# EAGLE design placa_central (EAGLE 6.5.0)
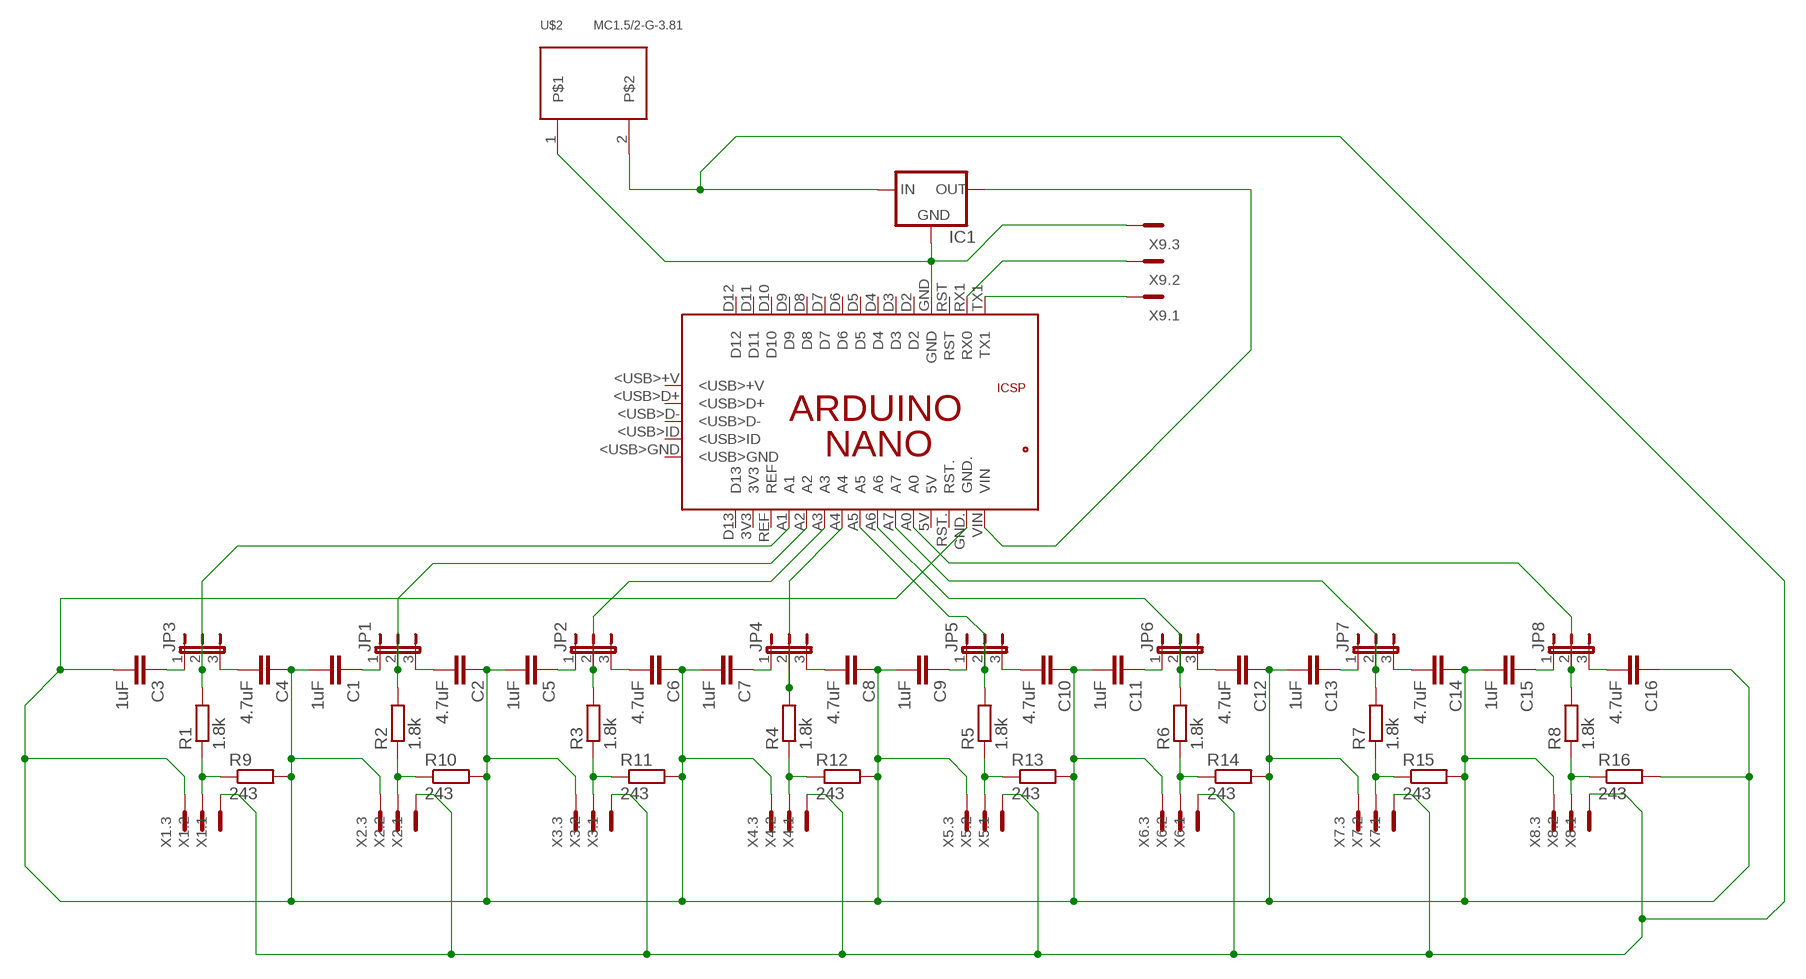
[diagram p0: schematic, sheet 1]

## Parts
C1  1uF  C-EUC1206  [C1206]
C2  4.7uF  C-EUC1206  [C1206]
C3  1uF  C-EUC1206  [C1206]
C4  4.7uF  C-EUC1206  [C1206]
C5  1uF  C-EUC1206  [C1206]
C6  4.7uF  C-EUC1206  [C1206]
C7  1uF  C-EUC1206  [C1206]
C8  4.7uF  C-EUC1206  [C1206]
C9  1uF  C-EUC1206  [C1206]
C10  4.7uF  C-EUC1206  [C1206]
C11  1uF  C-EUC1206  [C1206]
C12  4.7uF  C-EUC1206  [C1206]
C13  1uF  C-EUC1206  [C1206]
C14  4.7uF  C-EUC1206  [C1206]
C15  1uF  C-EUC1206  [C1206]
C16  4.7uF  C-EUC1206  [C1206]
IC1  78XXS  [78XXS]
JP1  JP2E  [JP2]
JP2  JP2E  [JP2]
JP3  JP2E  [JP2]
JP4  JP2E  [JP2]
JP5  JP2E  [JP2]
JP6  JP2E  [JP2]
JP7  JP2E  [JP2]
JP8  JP2E  [JP2]
PCB1  ARDUINO_NANO  [ARDUINO_NANO]
R1  1.8k  R-EU_M1206  [M1206]
R2  1.8k  R-EU_M1206  [M1206]
R3  1.8k  R-EU_M1206  [M1206]
R4  1.8k  R-EU_M1206  [M1206]
R5  1.8k  R-EU_M1206  [M1206]
R6  1.8k  R-EU_M1206  [M1206]
R7  1.8k  R-EU_M1206  [M1206]
R8  1.8k  R-EU_M1206  [M1206]
R9  243  R-EU_M1206  [M1206]
R10  243  R-EU_M1206  [M1206]
R11  243  R-EU_M1206  [M1206]
R12  243  R-EU_M1206  [M1206]
R13  243  R-EU_M1206  [M1206]
R14  243  R-EU_M1206  [M1206]
R15  243  R-EU_M1206  [M1206]
R16  243  R-EU_M1206  [M1206]
U$2  MC1.5/2-G-3.81  [MC1.5/2-G-3.81]
X1  MC3  [MC3]
X2  MC3  [MC3]
X3  MC3  [MC3]
X4  MC3  [MC3]
X5  MC3  [MC3]
X6  MC3  [MC3]
X7  MC3  [MC3]
X8  MC3  [MC3]
X9  MC3  [MC3]

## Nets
GND: C1.2 C2.1 C3.2 C4.1 C5.2 C6.1 C7.2 C8.1 C9.2 C10.1 C11.2 C12.1 C13.2 C14.1 C15.2 C16.1 IC1.GND PCB1.GND PCB1.GND. R9.2 R10.2 R11.2 R12.2 R13.2 R14.2 R15.2 R16.2 U$2.1 X1.3 X2.3 X3.3 X4.3 X5.3 X6.3 X7.3 X8.3 X9.3
N$1: R1.1 R9.1 X1.2
N$3: C4.2 JP3.3
N$4: C3.1 JP3.1
N$5: R2.1 R10.1 X2.2
N$6: PCB1.RX1(RX0) X9.2
N$7: C2.2 JP1.3
N$8: C1.1 JP1.1
N$9: R3.1 R11.1 X3.2
N$10: IC1.OUT PCB1.VIN
N$11: C6.2 JP2.3
N$12: C5.1 JP2.1
N$13: R4.1 R12.1 X4.2
N$14: PCB1.TX1 X9.1
N$15: C8.2 JP4.3
N$16: C7.1 JP4.1
N$17: R5.1 R13.1 X5.2
N$19: C10.2 JP5.3
N$20: C9.1 JP5.1
N$21: R6.1 R14.1 X6.2
N$23: C12.2 JP6.3
N$24: C11.1 JP6.1
N$25: R7.1 R15.1 X7.2
N$27: C14.2 JP7.3
N$28: C13.1 JP7.1
N$29: R8.1 R16.1 X8.2
N$31: C16.2 JP8.3
N$32: C15.1 JP8.1
N$33: JP3.2 PCB1.A1 R1.2
N$34: JP1.2 PCB1.A2 R2.2
N$35: JP2.2 PCB1.A3 R3.2
N$36: JP4.2 PCB1.A4 R4.2
N$37: JP8.2 PCB1.A0 R8.2
N$38: JP7.2 PCB1.A7 R7.2
N$39: JP6.2 PCB1.A6 R6.2
N$40: JP5.2 PCB1.A5 R5.2
N$59: IC1.IN U$2.2 X1.1 X2.1 X3.1 X4.1 X5.1 X6.1 X7.1 X8.1
Unconnected: PCB1.3V3 PCB1.5V PCB1.5V. PCB1.<USB>+V PCB1.<USB>D+ PCB1.<USB>D- PCB1.<USB>GND PCB1.<USB>ID PCB1.D2 PCB1.D3 PCB1.D4 PCB1.D5 PCB1.D6 PCB1.D7 PCB1.D8 PCB1.D9 PCB1.D10 PCB1.D11 PCB1.D12 PCB1.D13 PCB1.GND_ PCB1.MISO PCB1.MOSI PCB1.REF PCB1.RESET.. PCB1.RST PCB1.RST. PCB1.SCK

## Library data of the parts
C1-C16 = resistor:C-EU: CAPACITOR, European symbol
IC1 = v-reg:78XXS: VOLTAGE REGULATOR
JP1-JP8 = jumper:JP2E: JUMPER
PCB1 = E14_Arduino:ARDUINO_NANO: Device for representing an Arduino Nano board with a footprint in an EAGLE design. Created by Dave Young for Element14. More EAGLE documentation at: http://www.element14.com/community/community/knode/cadsoft_eagle
R1-R16 = resistor:R-EU_: RESISTOR, European symbol
U$2 = rpascoal:MC1.5/2-G-3.81
X1-X9 = con-phoenix-381_l:MC3: Mini-Combicon 3.81mm horizontal 3-polig (ohne Gegenstecker)

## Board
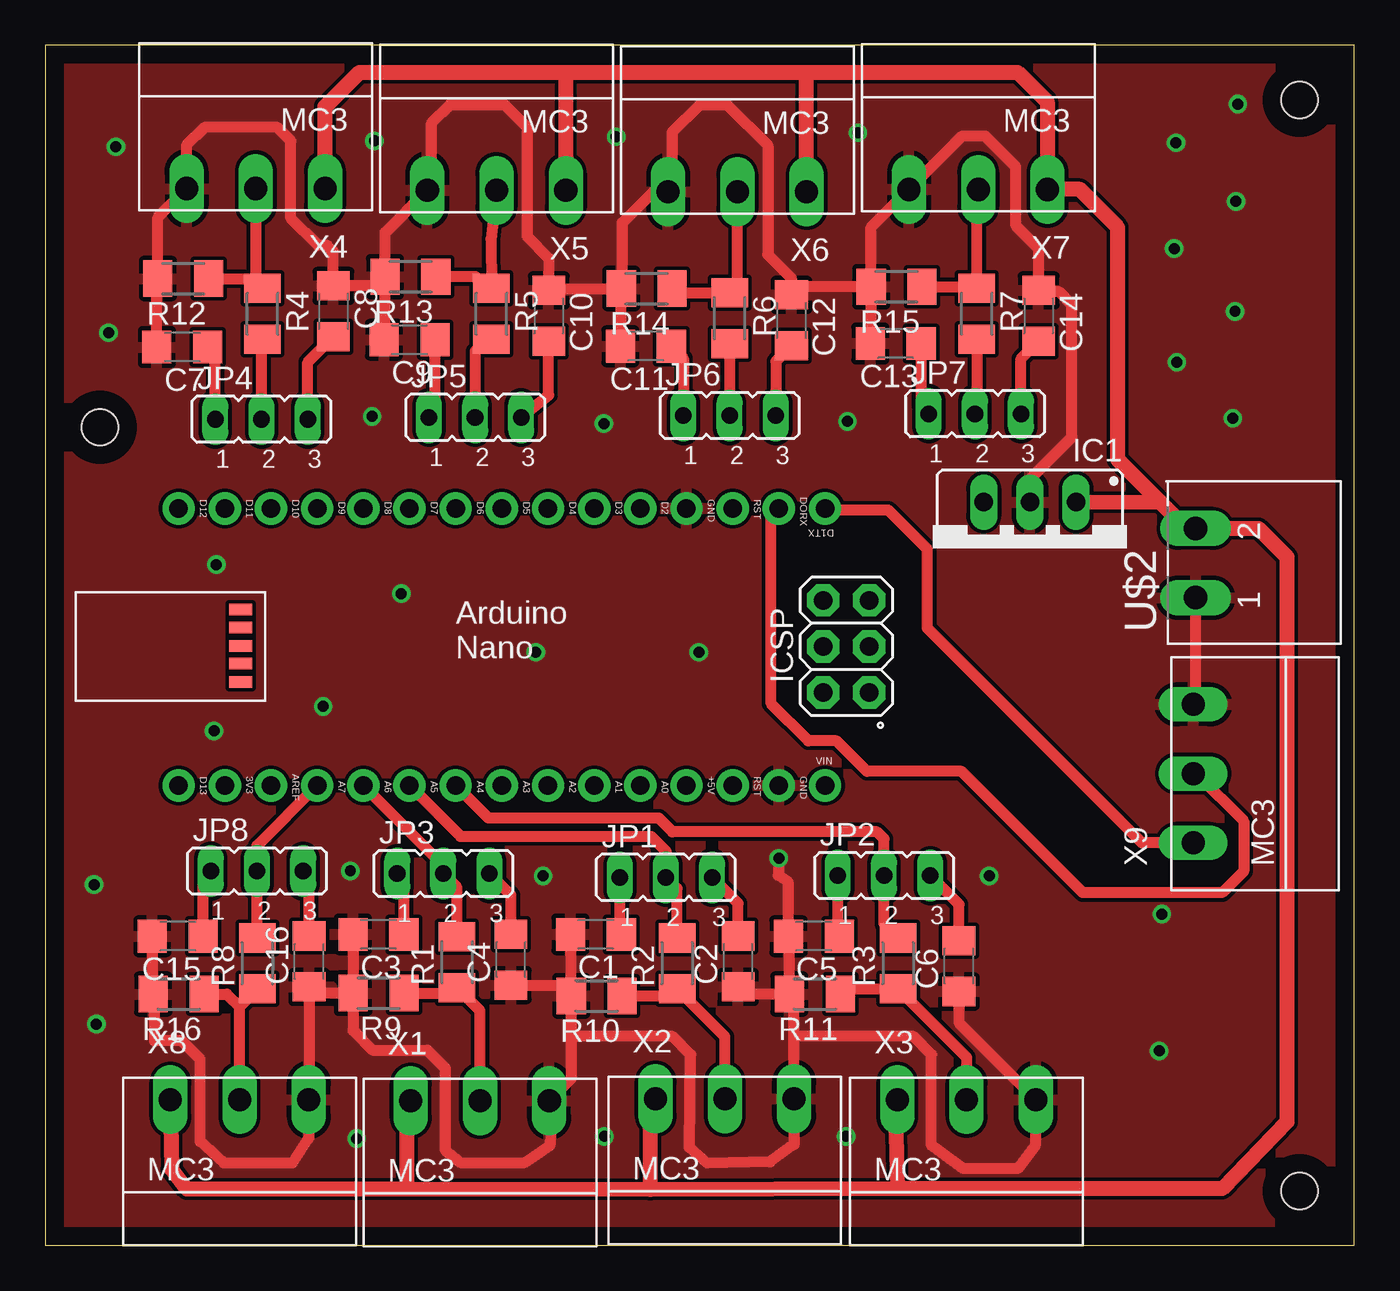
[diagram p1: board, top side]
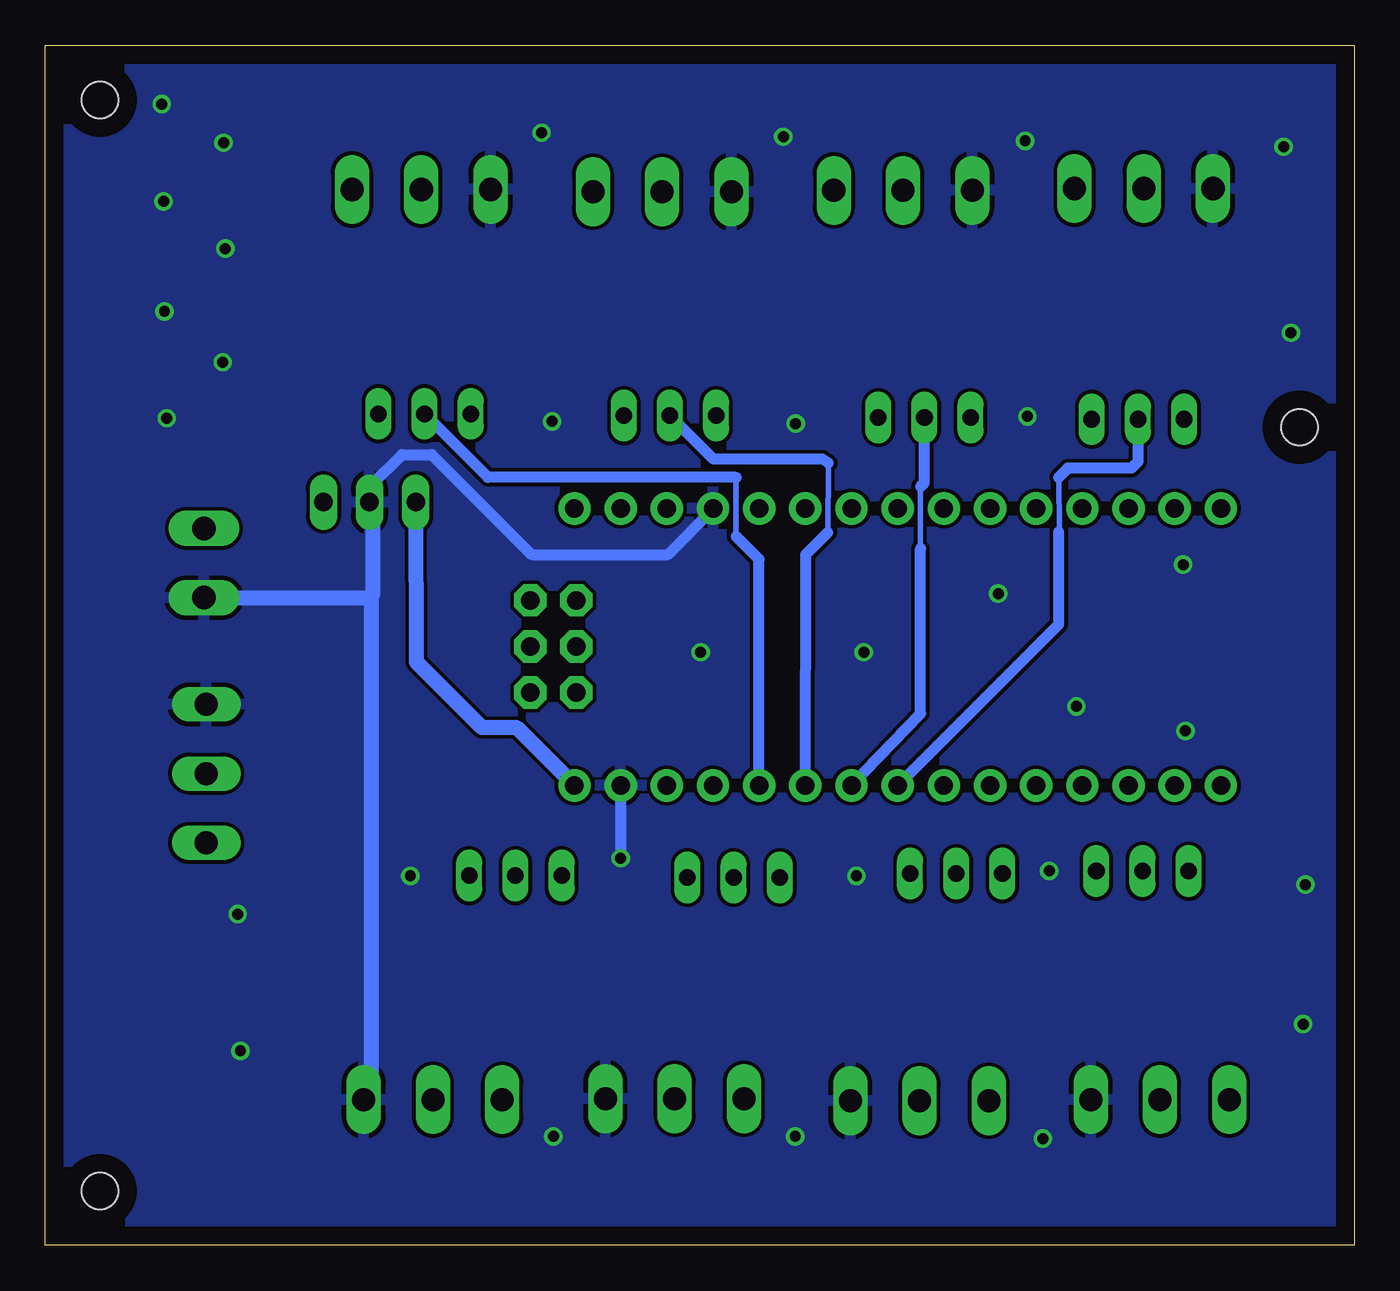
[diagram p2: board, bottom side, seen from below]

Size 72 x 66 mm. Coordinates in mm from the lower left corner, seen from the top.
Outline: 0,0 72,0 72,66 0,66 0,0
Copper layers (1*16): Top 0.035mm / dielectric 1.5mm / Bottom 0.035mm
Design rules "default": minimum track width 8mil, minimum drill 20mil, track to track 8mil, track to pad 8mil, pad to pad 8mil, via to via 10mil, smd to smd 8mil, copper to edge 40mil, drill to drill 8mil, minimum pad ring 10mil, minimum via ring 8mil, stop-mask expansion 4mil, vias tented up to drill 0mil, thermal gap 10mil
Holes 2 mm at 69,63 69,3 3,45

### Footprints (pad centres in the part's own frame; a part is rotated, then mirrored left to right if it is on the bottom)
C1206 = smd 1.6 x 1.8: 1 -1.4,0; 2 1.4,0
78XXS = drill 1.016 long: GND 0,-2.54; IN -2.54,-2.54; OUT 2.54,-2.54
JP2 = drill 0.914 long: 1 -2.54,0; 2 0,0; 3 2.54,0
ARDUINO_NANO = drill 1.016 pad 1.778: 3V3 6.35,1.27; 5V 31.75,1.27; A0 11.43,1.27; A1 13.97,1.27; A2 16.51,1.27; A3 19.05,1.27; A4 21.59,1.27; A5 24.13,1.27; A6 26.67,1.27; A7 29.21,1.27; D2 29.21,16.51; D3 26.67,16.51; D4 24.13,16.51; D5 21.59,16.51; D6 19.05,16.51; D7 16.51,16.51; D8 13.97,16.51; D9 11.43,16.51; D10 8.89,16.51; D11 6.35,16.51; D12 3.81,16.51; D13 3.81,1.27; GND 31.75,16.51; GND. 36.83,1.27; REF 8.89,1.27; RST 34.29,16.51; RST. 34.29,1.27; RX1 36.83,16.51; TX1 39.37,16.51; VIN 39.37,1.27 | drill 1.016 pad 1.778 octagon: 5V. 39.268,6.375; GND_ 39.268,11.455; MISO 41.808,6.375; MOSI 39.268,8.915; RESET.. 41.808,11.455; SCK 41.808,8.915 | smd 1.27 x 0.635: <USB>+V 7.214,10.947; <USB>D+ 7.214,9.957; <USB>D- 7.214,8.941; <USB>GND 7.214,6.96; <USB>ID 7.214,7.976
M1206 = smd 1.6 x 2: 1 -1.4,0; 2 1.4,0
MC1.5/2-G-3.81 = drill 1.3 long: 1 -3.81,8; 2 0,8
MC3 = drill 1.27 long: 1 -3.81,0; 2 0,0; 3 3.81,0

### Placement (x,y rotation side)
C1  30.28,17.11 180 top
C2  38.11,15.62 90 top
C3  18.32,17.11 180 top
C4  25.61,15.72 90 top
C5  42.28,17.01 180 top
C6  50.26,15.37 90 top
C7  7.53,49.41 180 top
C8  15.84,51.38 270 top
C9  20.03,49.81 180 top
C10  27.69,51.13 270 top
C11  33.03,49.46 180 top
C12  41.04,50.88 270 top
C13  46.78,49.61 180 top
C14  54.64,51.13 270 top
C15  7.28,17.01 180 top
C16  14.51,15.62 90 top
IC1  54.16,38.34 180 top
JP1  34.14,20.24 0 top
JP2  46.14,20.34 0 top
JP3  21.89,20.45 0 top
JP4  11.89,45.44 0 top
JP5  23.64,45.54 0 top
JP6  37.64,45.64 0 top
JP7  51.14,45.74 0 top
JP8  11.64,20.59 0 top
PCB1  3.52,24.03 0 top
R1  22.64,15.58 90 top
R2  34.76,15.51 90 top
R3  46.91,15.51 90 top
R4  11.94,51.24 270 top
R5  24.54,51.24 270 top
R6  37.64,50.99 270 top
R7  51.24,51.24 270 top
R8  11.66,15.51 90 top
R9  18.33,13.88 180 top
R10  30.33,13.73 180 top
R11  42.33,13.83 180 top
R12  7.58,53.18 180 top
R13  20.08,53.28 180 top
R14  33.08,52.63 180 top
R15  46.83,52.73 180 top
R16  7.33,13.83 180 top
U$2  71.28,39.44 90 top
X1  23.91,7.96 0 top
X2  37.38,8.07 0 top
X3  50.68,8.02 0 top
X4  11.57,58.13 180 top
X5  24.82,58.03 180 top
X6  38.07,57.95 180 top
X7  51.32,58.08 180 top
X8  10.68,8.02 0 top
X9  63.15,25.95 90 top

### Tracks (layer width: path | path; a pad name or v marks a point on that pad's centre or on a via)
GND  (via drill 0.6)
  Top 0.61: C15.2 5.88,13.88 R16.2 5.93,13.25 6,13.25 6,11.25 7.5,11.25 8.5,10.25 8.5,5.72 9.82,4.53 13.57,4.53 14.49,5.92 X8.3 14.51,9.79 C16.1 14.85,13.88 R9.2 | C3.2 R9.2 | R9.2 16.92,11.83 18,10.75 21,10.75 22,9.75 22,5.25 22.85,4.55 26.35,4.55 27.75,5.5 27.8,6.16 X1.3 28.93,9.18 28.93,11.25 | C1.2 28.88,13.78 R10.2 | R10.2 28.93,11.25 | 28.93,11.25 29.18,11.5 34.5,11.5 35.5,10.5 35.42,5.38 36.4,4.53 39.88,4.6 41.19,5.57 X2.3 41.19,11.5 | 41.19,11.5 41.19,13.57 R11.2 | R11.2 38.5,13.83 C2.1 | R11.2 40.93,16.96 C5.2 40.88,19.97 40.33,20.35 v40.35,21.3 | C4.1 28.34,14.32 R10.2 | 41.19,11.5 47.75,11.5 48.75,10.5 48.75,5.5 50.5,4.22 53.5,4.22 54.49,5.54 X3.3 50.26,12.25 C6.1 | C7.2 6.13,53.13 R12.2 6.18,56.55 X4.3 7.75,60.5 8.75,61.5 12.75,61.5 13.5,60.75 13.5,56.5 15,55 15.5,55 15.84,54.66 C8.1 18.18,52.78 R13.2 | C9.2 18.68,49.86 R13.2 | R13.2 18.68,55.7 X5.3 21.25,58.27 21.25,61.75 22.25,62.75 25.25,62.75 26.5,61.5 26.5,55.5 27.69,54.31 C10.1 27.79,52.63 R14.2 | R14.2 31.63,52.58 C11.2 | R14.2 31.75,52.7 31.75,56.25 33.68,58.18 X6.3 34.5,58.42 34.5,61.25 36,62.75 37.5,62.75 39.75,60.5 39.75,54.5 41.04,53.21 C12.1 41.49,52.73 R15.2 | R15.2 45.43,49.66 C13.2 | R15.2 45.43,56 X7.3 50.45,61.02 51.7,61.02 53.38,59.35 53.38,56.12 54.64,54.86 C14.1 54.72,52.45 55.77,52.45 56.48,51.75 56.48,44.45 54.14,42.12 IC1.GND | X9.3 63.28,29.76 U$2.1
  Bottom 0.61: PCB1.GND 35.27,40.48 37.75,38 45.25,38 50.75,43.5 52.39,43.5 54.14,41.75 IC1.GND | PCB1.GND. v40.35,21.3
  Bottom 0.813: U$2.1 54.15,35.63 54.05,35.73 | IC1.GND 54,40.76 54,35.77 54.05,35.73 | X3.3 54.05,8.46 54.05,35.73
  other vias: 65.6,62.77 65.5,57.42 65.45,51.38 65.33,45.5 62.25,48.58 62.1,54.83 62.2,60.65 61.42,18.23 61.27,10.7 15.28,29.65 19.57,35.85 35.95,32.62 26.98,32.62 9.4,37.45 9.28,28.3 3.88,60.42 3.48,50.2 2.67,19.85 2.8,12.18 44.12,45.33 30.73,45.2 17.98,45.6 27.38,20.32 16.77,20.6 51.92,20.32 44.05,6 30.75,6 17.12,5.88 44.7,61.2 31.4,60.98 18.1,60.75
  pour Bottom: 72.25,66.95 72.25,-0.57 -0.72,-0.57 -0.72,66.95
  pour Top: -1.18,67.7 72.97,67.7 72.97,-1.45 -1.6,-1.45
N$1
  Top 0.61: X1.2 23.91,12.91 R1.1 22.34,13.88 R9.1
N$3
  Top 0.61: C4.2 25.61,19.27 JP3.3
N$4
  Top 0.61: C3.1 19.72,20.08 JP3.1
N$5
  Top 0.61: X2.2 37.38,11.49 R2.1 34.38,13.73 R10.1
N$6
  Top 0.61: X9.2 63.33,25.95 65.92,23.35 65.92,20.57 64.75,19.4 57.08,19.4 50.4,26.07 45.2,26.07 43.52,27.75 41.98,27.75 39.92,29.8 39.92,40.12 PCB1.RX1
N$7
  Top 0.61: C2.2 38.11,18.81 JP1.3
N$8
  Top 0.61: C1.1 31.6,17.11 JP1.1
N$9
  Top 0.61: R11.1 44.01,14.11 R3.1 50.68,10.34 X3.2
N$10
  Bottom 0.813: IC1.OUT 51.6,32.1 48,28.5 46.09,28.5 PCB1.VIN
N$11
  Top 0.61: C6.2 50.26,18.76 JP2.3
N$12
  Top 0.61: C5.1 43.6,17.09 JP2.1
N$13
  Top 0.61: R12.1 11.4,53.18 R4.1 11.57,53.01 X4.2
N$14
  Top 0.61: X9.1 60.34,22.14 48.52,33.95 48.52,38.3 46.38,40.45 42.98,40.45 PCB1.TX1
N$15
  Top 0.61: JP4.3 14.43,48.57 C8.2
N$16
  Top 0.61: JP4.1 9.35,48.99 C7.1
N$17
  Top 0.61: X5.2 24.52,55.35 R5.1 23.65,53.28 R13.1
N$19
  Top 0.61: JP5.3 27.69,46.77 C10.2
N$20
  Top 0.61: JP5.1 21.43,45.87 C9.1
N$21
  Top 0.61: R14.1 34.72,52.39 R6.1 38.07,52.82 X6.2
N$23
  Top 0.61: C12.2 40.18,48.62 JP6.3
N$24
  Top 0.61: C11.1 35.1,48.79 JP6.1
N$25
  Top 0.61: R15.1 51.15,52.73 R7.1 51.24,58 X7.2
N$27
  Top 0.61: JP7.3 53.68,48.77 C14.2
N$28
  Top 0.61: C13.1 48.18,46.16 JP7.1
N$29
  Top 0.61: X8.2 10.68,13.13 | 10.68,13.13 R8.1 | R16.1 9.98,13.83 10.68,13.13
N$31
  Top 0.61: C16.2 14.51,20.26 JP8.3
N$32
  Top 0.61: C15.1 8.68,20.17 JP8.1
N$33
  Top 0.61: R1.2 22.64,19.7 JP3.2 21.89,20.9 PCB1.A1
N$34
  Top 0.61: R2.2 34.76,19.62 JP1.2 34.14,21.66 34.15,21.68 33.33,22.5 22.83,22.5 PCB1.A2
N$35
  Top 0.61: R3.2 46.14,17.68 JP2.2 46.14,22.36 45.75,22.75 34.5,22.75 33.75,23.5 24.37,23.5 PCB1.A3
N$36
  Top 0.61: JP4.2 11.89,49.79 R4.2
  Bottom 0.305: 16.23,39.27 16.25,42.25
  Bottom 0.406: 16.25,39.25 16.23,39.27
  Bottom 0.61: PCB1.A4 16.25,34.16 16.25,39.25 | JP4.2 11.89,43.11 12.25,42.75 15.75,42.75 16.25,42.25
N$37
  Top 0.61: R8.2 11.66,20.57 JP8.2 11.64,21.99 PCB1.A0
N$38
  Top 0.61: R7.2 51.24,45.84 JP7.2
  Bottom 0.305: 34,39 34,42.25
  Bottom 0.61: PCB1.A7 32.73,37.73 34,39 | 34,42.25 47.65,42.25 JP7.2
N$39
  Top 0.61: R6.2 JP6.2
  Bottom 0.305: 28.95,39.23 28.93,43.02
  Bottom 0.61: PCB1.A6 30.16,38.01 28.95,39.23 | 28.93,43.02 29.25,43.25 35.25,43.25 JP6.2
N$40
  Top 0.61: R5.2 23.64,49.19 JP5.2
  Bottom 0.305: 23.85,38.38 23.85,41.75
  Bottom 0.406: 23.85,38.33 23.85,38.38
  Bottom 0.61: PCB1.A5 23.85,29.25 23.85,38.33 | 23.85,41.75 23.64,41.94 JP5.2
N$59
  Top 0.813: 6.73,8.02 X8.1 6.95,4.18 7.78,3.1 19.88,3.1 | 61.32,40.9 59,43.22 59,56 56.92,58.08 X7.1 55.12,62.9 53.5,64.53 41.92,64.53 | IC1.IN 61.32,40.9 | 61.32,40.9 62.78,39.44 U$2.2 66.73,39.44 68.3,37.88 68.3,6.8 64.75,3.12 46.88,3.12 | 46.88,3.12 33.27,3.08 | 33.27,3.08 19.88,3.1 | X1.1 19.88,7.96 19.88,3.1 | X2.1 33.25,8.07 33.27,3.08 | X3.1 46.73,8.02 46.88,3.12 | X4.1 15.38,62.63 17.27,64.53 28.65,64.53 | 28.65,64.53 41.92,64.53 | X5.1 28.63,64.5 28.65,64.53 | X6.1 41.88,64.48 41.92,64.53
